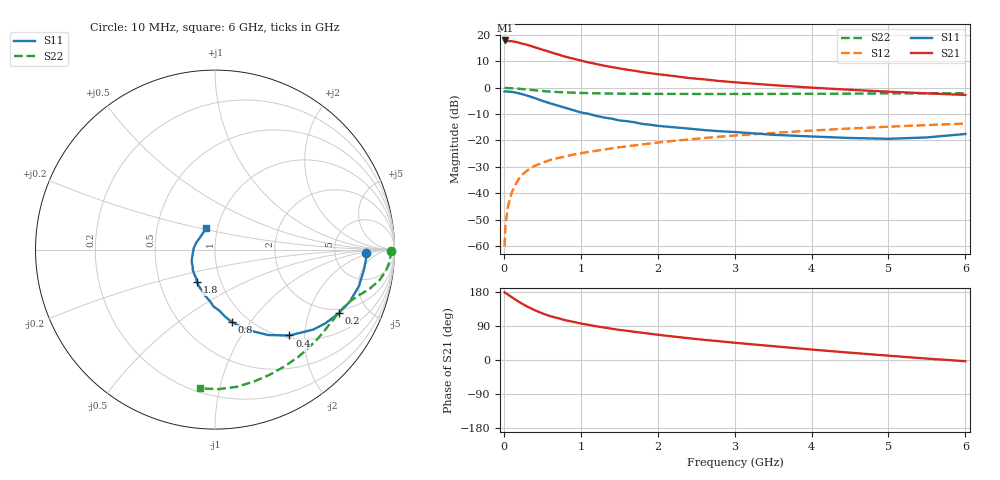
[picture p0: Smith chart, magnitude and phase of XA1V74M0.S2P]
! SIEMENS Discrete & RF Semiconductors
! BFY180
! Si NPN RF Bipolar Junction Transistor in MICRO-X
! VCE = 1.75 V  IC = 4 mA
! Common Emitter S-Parameters:  May  1997
# GHz  S  MA  R  50
!  f  S11  S21  S12  S22
! GHz  MAG  ANG  MAG  ANG  MAG  ANG  MAG  ANG
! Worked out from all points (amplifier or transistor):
!   36 points, 10 MHz to 6 GHz, reference 50 ohm
!   highest |S21| = 17.8 dB at 20 MHz (marker M1)
!   |S21| within 3 dB of that: start of sweep to 450.2 MHz
!   unconditionally stable (mu >= 1): 950.3 MHz to end of sweep
!   at 250 MHz: K = 0.35, MSG = 24.6 dB, |S12| = -32.7 dB
!   at 1.4 GHz: K = 1.20, MAG = 12.7 dB, |S12| = -23.0 dB
!   at 6 GHz: K = 1.26, MAG = 2.4 dB, |S12| = -13.6 dB
!   S11 on the Smith chart (normalised r, x): 10 MHz: 11, -2; 200 MHz: 1.79, -3.18; 400 MHz: 1.05, -1.67; 800 MHz: 0.84, -0.82; 1.8 GHz: 0.77, -0.29; 6 GHz: 0.88, +0.22
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0.01  0.8421 -1.4  7.633 178.6  0.001 81.0  0.9796 -0.3
0.02  0.8448 -2.7  7.768 176.9  0.0024 91.6  0.9855 -0.9
0.05  0.8382 -7.2  7.575 173.2  0.0053 85.7  0.9779 -2.3
0.1  0.8278 -14.1  7.521 166.2  0.0101 81.6  0.9717 -4.6
0.15  0.8051 -21.1  7.304 159.4  0.0146 78.6  0.9616 -6.7
0.2  0.7746 -27.3  7.027 153.0  0.0191 73.6  0.9472 -8.6
0.25  0.7404 -33.6  6.708 147.1  0.0232 71.8  0.9333 -10.4
0.3  0.7063 -39.1  6.444 141.4  0.0267 68.5  0.9163 -11.8
0.4  0.6328 -49.1  5.799 131.7  0.033 64.7  0.8878 -14.3
0.5  0.5608 -58.1  5.217 123.1  0.0377 60.7  0.8602 -16.2
0.6  0.5033 -64.9  4.692 115.8  0.0425 59.1  0.839 -17.8
0.8  0.4136 -77.1  3.828 105.0  0.0498 56.3  0.8086 -20.6
1  0.3386 -86.3  3.238 96.4  0.0571 54.7  0.7905 -23.4
1.1  0.3184 -91.2  2.992 92.7  0.0605 54.3  0.7832 -24.6
1.4  0.2585 -103.7  2.442 82.5  0.0705 52.9  0.7691 -28.8
1.8  0.2049 -119.1  1.959 71.8  0.084 51.6  0.76 -34.5
2.2  0.1778 -130.9  1.656 62.0  0.0979 49.3  0.7578 -40.5
2.8  0.1494 -149.3  1.33 49.5  0.1174 45.8  0.7559 -49.2
3.5  0.1278 -167.9  1.11 36.5  0.1386 40.8  0.7573 -59.2
4.5  0.1111 159.2  0.907 19.3  0.1678 33.4  0.7663 -73.6
5.5  0.1139 125.8  0.776 3.7  0.195 25.5  0.7776 -88.6
6  0.1323 111.6  0.724 -3.2  0.208 21.2  0.7781 -96.2
